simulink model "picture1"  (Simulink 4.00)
settings: Solver=ode45  StartTime=0.0  StopTime=10.0  RelTol=1e-3
undefined symbols (not defined in the file or in its folder): Kd, Kg, Ktg, Ku, Tg, Tja, Tm

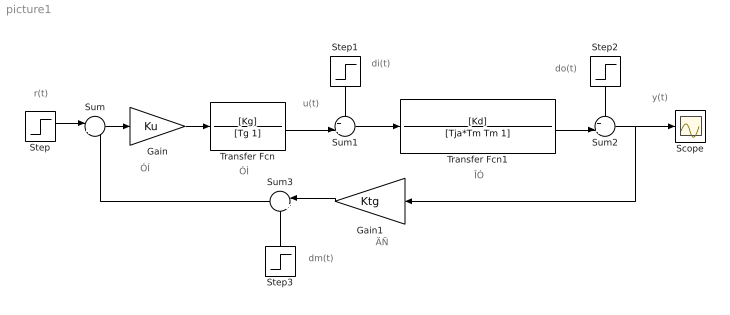
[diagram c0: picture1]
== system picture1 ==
  note: r(t)
  note: u(t)
  note: y(t)
  note: di(t)
  note: do(t)
  note: dm(t)
  note: ÓÍ
  note: ÓÌ
  note: ÎÓ
  note: ÄÑ
  Gain : Gain  Gain=Ku  Multiplication=Element-wise(K.*u)  SaturateOnIntegerOverflow=on
  Gain1 : Gain  Orientation=left  Gain=Ktg  Multiplication=Element-wise(K.*u)  SaturateOnIntegerOverflow=on
  Scope : Scope
  Step : Step  Time=1  Before=0  After=1  SampleTime=0
  Step1 : Step  Orientation=down  Time=3  Before=0  After=-.1  SampleTime=0
  Step2 : Step  Orientation=down  Time=6  Before=0  After=-.1  SampleTime=0
  Step3 : Step  Orientation=up  Time=9  Before=0  After=-.1  SampleTime=0
  Sum : Sum  Inputs=|+-  SaturateOnIntegerOverflow=on
  Sum1 : Sum  Inputs=++|  SaturateOnIntegerOverflow=on
  Sum2 : Sum  Inputs=++|  SaturateOnIntegerOverflow=on
  Sum3 : Sum  Orientation=left  Inputs=|++  SaturateOnIntegerOverflow=on
  Transfer Fcn : TransferFcn  Numerator=[Kg]  Denominator=[Tg 1]  AbsoluteTolerance=auto  Realization=auto
  Transfer Fcn1 : TransferFcn  Numerator=[Kd]  Denominator=[Tja*Tm Tm 1]  AbsoluteTolerance=auto  Realization=auto
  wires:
  Gain/1 -> Transfer Fcn/1
  Step/1 -> Sum/1
  Sum/1 -> Gain/1
  Step1/1 -> Sum1/1
  Transfer Fcn/1 -> Sum1/2
  Sum1/1 -> Transfer Fcn1/1
  Step2/1 -> Sum2/1
  Transfer Fcn1/1 -> Sum2/2
  Sum2/1 -> Scope/1, Gain1/1
  Sum3/1 -> Sum/2
  Step3/1 -> Sum3/2
  Gain1/1 -> Sum3/1
